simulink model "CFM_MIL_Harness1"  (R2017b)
settings: Solver=FixedStepDiscrete  StartTime=0.0  StopTime=14  FixedStep=0.01  RelTol=1e-3  EnableMultiTasking=on
undefined symbols (not defined in the file): sigbuilder_block
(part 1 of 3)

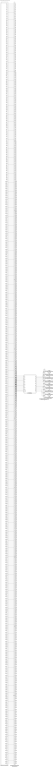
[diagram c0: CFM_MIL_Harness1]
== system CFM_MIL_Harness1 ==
  CFM_MIL : ModelReference  ModelNameDialog=CFM_MIL  SimulationMode=Normal  ModelReferenceVersion='M103C102'
  Harness Inputs : Subsystem  Tag=STV Subsys  LoadFcn=sigbuilder_block('load');  StartFcn=sigbuilder_block('start');  StopFcn=sigbuilder_block('stop');  ClipboardFcn=sigbuilder_block('clipboard');  mask(Sigbuilder block){tuvar=[0:10]}
      mask init:
      | if ~strcmp(get_param(bdroot(gcb),'SimulationStatus'),'stopped'),tuvar = sigbuilder_block('maskInit'); end
  Input Conversion Subsystem : Subsystem  Tag=__SLT_ICS__  Description=Signal spec. and routing
  Output Conversion Subsystem : Subsystem  Tag=__SLT_OCS__  Description=Signal spec. and routing
  GaCFM_AFEComLost_flg : Outport  OutDataTypeStr=boolean  PortDimensions=[8]
  GaCFM_AFECellVoltUpdErr_flg : Outport  Port=2  OutDataTypeStr=boolean  PortDimensions=[8]
  GaCFM_AFECellTempUpdErr_flg : Outport  Port=3  OutDataTypeStr=boolean  PortDimensions=[8]
  GaCFM_AFECellVoltLineOpen_flg : Outport  Port=4  OutDataTypeStr=boolean  PortDimensions=[8]
  GaCFM_AFEGpioLineOpen_flg : Outport  Port=5  OutDataTypeStr=boolean  PortDimensions=[8]
  GaCFM_AFEAdcRelatedErr_flg : Outport  Port=6  OutDataTypeStr=boolean  PortDimensions=[8]
  GaCFM_AFEDiagModeExitErr_flg : Outport  Port=7  OutDataTypeStr=boolean  PortDimensions=[8]
  GaCFM_AFEOtherErr_flg : Outport  Port=8  OutDataTypeStr=boolean  PortDimensions=[8]
  GaCFM_AFESampleErr_flg : Outport  Port=9  OutDataTypeStr=boolean  PortDimensions=[8]
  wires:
  Harness Inputs/1(GaISP_AFEComLost_numb(1)) -> Input Conversion Subsystem/1(Inport_1)
  Harness Inputs/2(GaISP_AFEComLost_numb(2)) -> Input Conversion Subsystem/2(Inport_2)
  Harness Inputs/3(GaISP_AFEComLost_numb(3)) -> Input Conversion Subsystem/3(Inport_3)
  Harness Inputs/4(GaISP_AFEComLost_numb(4)) -> Input Conversion Subsystem/4(Inport_4)
  Harness Inputs/5(GaISP_AFEComLost_numb(5)) -> Input Conversion Subsystem/5(Inport_5)
  Harness Inputs/6(GaISP_AFEComLost_numb(6)) -> Input Conversion Subsystem/6(Inport_6)
  Harness Inputs/7(GaISP_AFEComLost_numb(7)) -> Input Conversion Subsystem/7(Inport_7)
  Harness Inputs/8(GaISP_AFEComLost_numb(8)) -> Input Conversion Subsystem/8(Inport_8)
  Harness Inputs/9(GaISP_AFECellVoltUpdErr_numb(1)) -> Input Conversion Subsystem/9(Inport_9)
  Harness Inputs/10(GaISP_AFECellVoltUpdErr_numb(2)) -> Input Conversion Subsystem/10(Inport_10)
  Harness Inputs/11(GaISP_AFECellVoltUpdErr_numb(3)) -> Input Conversion Subsystem/11(Inport_11)
  Harness Inputs/12(GaISP_AFECellVoltUpdErr_numb(4)) -> Input Conversion Subsystem/12(Inport_12)
  Harness Inputs/13(GaISP_AFECellVoltUpdErr_numb(5)) -> Input Conversion Subsystem/13(Inport_13)
  Harness Inputs/14(GaISP_AFECellVoltUpdErr_numb(6)) -> Input Conversion Subsystem/14(Inport_14)
  Harness Inputs/15(GaISP_AFECellVoltUpdErr_numb(7)) -> Input Conversion Subsystem/15(Inport_15)
  Harness Inputs/16(GaISP_AFECellVoltUpdErr_numb(8)) -> Input Conversion Subsystem/16(Inport_16)
  Harness Inputs/17(GaISP_AFECellVoltUpdErr_numb(9)) -> Input Conversion Subsystem/17(Inport_17)
  Harness Inputs/18(GaISP_AFECellVoltUpdErr_numb(10)) -> Input Conversion Subsystem/18(Inport_18)
  Harness Inputs/19(GaISP_AFECellVoltUpdErr_numb(11)) -> Input Conversion Subsystem/19(Inport_19)
  Harness Inputs/20(GaISP_AFECellVoltUpdErr_numb(12)) -> Input Conversion Subsystem/20(Inport_20)
  Harness Inputs/21(GaISP_AFECellVoltUpdErr_numb(13)) -> Input Conversion Subsystem/21(Inport_21)
  Harness Inputs/22(GaISP_AFECellVoltUpdErr_numb(14)) -> Input Conversion Subsystem/22(Inport_22)
  Harness Inputs/23(GaISP_AFECellVoltUpdErr_numb(15)) -> Input Conversion Subsystem/23(Inport_23)
  Harness Inputs/24(GaISP_AFECellVoltUpdErr_numb(16)) -> Input Conversion Subsystem/24(Inport_24)
  Harness Inputs/25(GaISP_AFECellVoltUpdErr_numb(17)) -> Input Conversion Subsystem/25(Inport_25)
  Harness Inputs/26(GaISP_AFECellVoltUpdErr_numb(18)) -> Input Conversion Subsystem/26(Inport_26)
  Harness Inputs/27(GaISP_AFECellVoltUpdErr_numb(19)) -> Input Conversion Subsystem/27(Inport_27)
  Harness Inputs/28(GaISP_AFECellVoltUpdErr_numb(20)) -> Input Conversion Subsystem/28(Inport_28)
  Harness Inputs/29(GaISP_AFECellVoltUpdErr_numb(21)) -> Input Conversion Subsystem/29(Inport_29)
  Harness Inputs/30(GaISP_AFECellVoltUpdErr_numb(22)) -> Input Conversion Subsystem/30(Inport_30)
  Harness Inputs/31(GaISP_AFECellVoltUpdErr_numb(23)) -> Input Conversion Subsystem/31(Inport_31)
  Harness Inputs/32(GaISP_AFECellVoltUpdErr_numb(24)) -> Input Conversion Subsystem/32(Inport_32)
  Harness Inputs/33(GaISP_AFECellVoltUpdErr_numb(25)) -> Input Conversion Subsystem/33(Inport_33)
  Harness Inputs/34(GaISP_AFECellVoltUpdErr_numb(26)) -> Input Conversion Subsystem/34(Inport_34)
  Harness Inputs/35(GaISP_AFECellVoltUpdErr_numb(27)) -> Input Conversion Subsystem/35(Inport_35)
  Harness Inputs/36(GaISP_AFECellVoltUpdErr_numb(28)) -> Input Conversion Subsystem/36(Inport_36)
  Harness Inputs/37(GaISP_AFECellVoltUpdErr_numb(29)) -> Input Conversion Subsystem/37(Inport_37)
  Harness Inputs/38(GaISP_AFECellVoltUpdErr_numb(30)) -> Input Conversion Subsystem/38(Inport_38)
  Harness Inputs/39(GaISP_AFECellVoltUpdErr_numb(31)) -> Input Conversion Subsystem/39(Inport_39)
  Harness Inputs/40(GaISP_AFECellVoltUpdErr_numb(32)) -> Input Conversion Subsystem/40(Inport_40)
  Harness Inputs/41(GaISP_AFECellVoltUpdErr_numb(33)) -> Input Conversion Subsystem/41(Inport_41)
  Harness Inputs/42(GaISP_AFECellVoltUpdErr_numb(34)) -> Input Conversion Subsystem/42(Inport_42)
  Harness Inputs/43(GaISP_AFECellVoltUpdErr_numb(35)) -> Input Conversion Subsystem/43(Inport_43)
  Harness Inputs/44(GaISP_AFECellVoltUpdErr_numb(36)) -> Input Conversion Subsystem/44(Inport_44)
  Harness Inputs/45(GaISP_AFECellVoltUpdErr_numb(37)) -> Input Conversion Subsystem/45(Inport_45)
  Harness Inputs/46(GaISP_AFECellVoltUpdErr_numb(38)) -> Input Conversion Subsystem/46(Inport_46)
  Harness Inputs/47(GaISP_AFECellVoltUpdErr_numb(39)) -> Input Conversion Subsystem/47(Inport_47)
  Harness Inputs/48(GaISP_AFECellVoltUpdErr_numb(40)) -> Input Conversion Subsystem/48(Inport_48)
  Harness Inputs/49(GaISP_AFECellVoltUpdErr_numb(41)) -> Input Conversion Subsystem/49(Inport_49)
  Harness Inputs/50(GaISP_AFECellVoltUpdErr_numb(42)) -> Input Conversion Subsystem/50(Inport_50)
  Harness Inputs/51(GaISP_AFECellVoltUpdErr_numb(43)) -> Input Conversion Subsystem/51(Inport_51)
  Harness Inputs/52(GaISP_AFECellVoltUpdErr_numb(44)) -> Input Conversion Subsystem/52(Inport_52)
  Harness Inputs/53(GaISP_AFECellVoltUpdErr_numb(45)) -> Input Conversion Subsystem/53(Inport_53)
  Harness Inputs/54(GaISP_AFECellVoltUpdErr_numb(46)) -> Input Conversion Subsystem/54(Inport_54)
  Harness Inputs/55(GaISP_AFECellVoltUpdErr_numb(47)) -> Input Conversion Subsystem/55(Inport_55)
  Harness Inputs/56(GaISP_AFECellVoltUpdErr_numb(48)) -> Input Conversion Subsystem/56(Inport_56)
  Harness Inputs/57(GaISP_AFECellVoltUpdErr_numb(49)) -> Input Conversion Subsystem/57(Inport_57)
  Harness Inputs/58(GaISP_AFECellVoltUpdErr_numb(50)) -> Input Conversion Subsystem/58(Inport_58)
  Harness Inputs/59(GaISP_AFECellVoltUpdErr_numb(51)) -> Input Conversion Subsystem/59(Inport_59)
  Harness Inputs/60(GaISP_AFECellVoltUpdErr_numb(52)) -> Input Conversion Subsystem/60(Inport_60)
  Harness Inputs/61(GaISP_AFECellVoltUpdErr_numb(53)) -> Input Conversion Subsystem/61(Inport_61)
  Harness Inputs/62(GaISP_AFECellVoltUpdErr_numb(54)) -> Input Conversion Subsystem/62(Inport_62)
  Harness Inputs/63(GaISP_AFECellVoltUpdErr_numb(55)) -> Input Conversion Subsystem/63(Inport_63)
  Harness Inputs/64(GaISP_AFECellVoltUpdErr_numb(56)) -> Input Conversion Subsystem/64(Inport_64)
  Harness Inputs/65(GaISP_AFECellVoltUpdErr_numb(57)) -> Input Conversion Subsystem/65(Inport_65)
  Harness Inputs/66(GaISP_AFECellVoltUpdErr_numb(58)) -> Input Conversion Subsystem/66(Inport_66)
  Harness Inputs/67(GaISP_AFECellVoltUpdErr_numb(59)) -> Input Conversion Subsystem/67(Inport_67)
  Harness Inputs/68(GaISP_AFECellVoltUpdErr_numb(60)) -> Input Conversion Subsystem/68(Inport_68)
  Harness Inputs/69(GaISP_AFECellVoltUpdErr_numb(61)) -> Input Conversion Subsystem/69(Inport_69)
  Harness Inputs/70(GaISP_AFECellVoltUpdErr_numb(62)) -> Input Conversion Subsystem/70(Inport_70)
  Harness Inputs/71(GaISP_AFECellVoltUpdErr_numb(63)) -> Input Conversion Subsystem/71(Inport_71)
  Harness Inputs/72(GaISP_AFECellVoltUpdErr_numb(64)) -> Input Conversion Subsystem/72(Inport_72)
  Harness Inputs/73(GaISP_AFECellVoltUpdErr_numb(65)) -> Input Conversion Subsystem/73(Inport_73)
  Harness Inputs/74(GaISP_AFECellVoltUpdErr_numb(66)) -> Input Conversion Subsystem/74(Inport_74)
  Harness Inputs/75(GaISP_AFECellVoltUpdErr_numb(67)) -> Input Conversion Subsystem/75(Inport_75)
  Harness Inputs/76(GaISP_AFECellVoltUpdErr_numb(68)) -> Input Conversion Subsystem/76(Inport_76)
  Harness Inputs/77(GaISP_AFECellVoltUpdErr_numb(69)) -> Input Conversion Subsystem/77(Inport_77)
  Harness Inputs/78(GaISP_AFECellVoltUpdErr_numb(70)) -> Input Conversion Subsystem/78(Inport_78)
  Harness Inputs/79(GaISP_AFECellVoltUpdErr_numb(71)) -> Input Conversion Subsystem/79(Inport_79)
  Harness Inputs/80(GaISP_AFECellVoltUpdErr_numb(72)) -> Input Conversion Subsystem/80(Inport_80)
  Harness Inputs/81(GaISP_AFECellVoltUpdErr_numb(73)) -> Input Conversion Subsystem/81(Inport_81)
  Harness Inputs/82(GaISP_AFECellVoltUpdErr_numb(74)) -> Input Conversion Subsystem/82(Inport_82)
  Harness Inputs/83(GaISP_AFECellVoltUpdErr_numb(75)) -> Input Conversion Subsystem/83(Inport_83)
  Harness Inputs/84(GaISP_AFECellVoltUpdErr_numb(76)) -> Input Conversion Subsystem/84(Inport_84)
  Harness Inputs/85(GaISP_AFECellVoltUpdErr_numb(77)) -> Input Conversion Subsystem/85(Inport_85)
  Harness Inputs/86(GaISP_AFECellVoltUpdErr_numb(78)) -> Input Conversion Subsystem/86(Inport_86)
  Harness Inputs/87(GaISP_AFECellVoltUpdErr_numb(79)) -> Input Conversion Subsystem/87(Inport_87)
  Harness Inputs/88(GaISP_AFECellVoltUpdErr_numb(80)) -> Input Conversion Subsystem/88(Inport_88)
  Harness Inputs/89(GaISP_AFECellVoltUpdErr_numb(81)) -> Input Conversion Subsystem/89(Inport_89)
  Harness Inputs/90(GaISP_AFECellVoltUpdErr_numb(82)) -> Input Conversion Subsystem/90(Inport_90)
  Harness Inputs/91(GaISP_AFECellVoltUpdErr_numb(83)) -> Input Conversion Subsystem/91(Inport_91)
  Harness Inputs/92(GaISP_AFECellVoltUpdErr_numb(84)) -> Input Conversion Subsystem/92(Inport_92)
  Harness Inputs/93(GaISP_AFECellVoltUpdErr_numb(85)) -> Input Conversion Subsystem/93(Inport_93)
  Harness Inputs/94(GaISP_AFECellVoltUpdErr_numb(86)) -> Input Conversion Subsystem/94(Inport_94)
  Harness Inputs/95(GaISP_AFECellVoltUpdErr_numb(87)) -> Input Conversion Subsystem/95(Inport_95)
  Harness Inputs/96(GaISP_AFECellVoltUpdErr_numb(88)) -> Input Conversion Subsystem/96(Inport_96)
  Harness Inputs/97(GaISP_AFECellVoltUpdErr_numb(89)) -> Input Conversion Subsystem/97(Inport_97)
  Harness Inputs/98(GaISP_AFECellVoltUpdErr_numb(90)) -> Input Conversion Subsystem/98(Inport_98)
  Harness Inputs/99(GaISP_AFECellVoltUpdErr_numb(91)) -> Input Conversion Subsystem/99(Inport_99)
  Harness Inputs/100(GaISP_AFECellVoltUpdErr_numb(92)) -> Input Conversion Subsystem/100(Inport_100)
  Harness Inputs/101(GaISP_AFECellVoltUpdErr_numb(93)) -> Input Conversion Subsystem/101(Inport_101)
  Harness Inputs/102(GaISP_AFECellVoltUpdErr_numb(94)) -> Input Conversion Subsystem/102(Inport_102)
  Harness Inputs/103(GaISP_AFECellVoltUpdErr_numb(95)) -> Input Conversion Subsystem/103(Inport_103)
  Harness Inputs/104(GaISP_AFECellVoltUpdErr_numb(96)) -> Input Conversion Subsystem/104(Inport_104)
  Harness Inputs/105(GaISP_AFECellVoltUpdErr_numb(97)) -> Input Conversion Subsystem/105(Inport_105)
  Harness Inputs/106(GaISP_AFECellVoltUpdErr_numb(98)) -> Input Conversion Subsystem/106(Inport_106)
  Harness Inputs/107(GaISP_AFECellVoltUpdErr_numb(99)) -> Input Conversion Subsystem/107(Inport_107)
  Harness Inputs/108(GaISP_AFECellVoltUpdErr_numb(100)) -> Input Conversion Subsystem/108(Inport_108)
  Harness Inputs/109(GaISP_AFECellVoltUpdErr_numb(101)) -> Input Conversion Subsystem/109(Inport_109)
  Harness Inputs/110(GaISP_AFECellVoltUpdErr_numb(102)) -> Input Conversion Subsystem/110(Inport_110)
  Harness Inputs/111(GaISP_AFECellVoltUpdErr_numb(103)) -> Input Conversion Subsystem/111(Inport_111)
  Harness Inputs/112(GaISP_AFECellVoltUpdErr_numb(104)) -> Input Conversion Subsystem/112(Inport_112)
  Harness Inputs/113(GaISP_AFECellVoltUpdErr_numb(105)) -> Input Conversion Subsystem/113(Inport_113)
  Harness Inputs/114(GaISP_AFECellVoltUpdErr_numb(106)) -> Input Conversion Subsystem/114(Inport_114)
  Harness Inputs/115(GaISP_AFECellVoltUpdErr_numb(107)) -> Input Conversion Subsystem/115(Inport_115)
  Harness Inputs/116(GaISP_AFECellVoltUpdErr_numb(108)) -> Input Conversion Subsystem/116(Inport_116)
  Harness Inputs/117(GaISP_AFECellVoltUpdErr_numb(109)) -> Input Conversion Subsystem/117(Inport_117)
  Harness Inputs/118(GaISP_AFECellVoltUpdErr_numb(110)) -> Input Conversion Subsystem/118(Inport_118)
  Harness Inputs/119(GaISP_AFECellVoltUpdErr_numb(111)) -> Input Conversion Subsystem/119(Inport_119)
  Harness Inputs/120(GaISP_AFECellVoltUpdErr_numb(112)) -> Input Conversion Subsystem/120(Inport_120)
  Harness Inputs/121(GaISP_AFECellTempUpdErr_numb(1)) -> Input Conversion Subsystem/121(Inport_121)
  Harness Inputs/122(GaISP_AFECellTempUpdErr_numb(2)) -> Input Conversion Subsystem/122(Inport_122)
  Harness Inputs/123(GaISP_AFECellTempUpdErr_numb(3)) -> Input Conversion Subsystem/123(Inport_123)
  Harness Inputs/124(GaISP_AFECellTempUpdErr_numb(4)) -> Input Conversion Subsystem/124(Inport_124)
  Harness Inputs/125(GaISP_AFECellTempUpdErr_numb(5)) -> Input Conversion Subsystem/125(Inport_125)
  Harness Inputs/126(GaISP_AFECellTempUpdErr_numb(6)) -> Input Conversion Subsystem/126(Inport_126)
  Harness Inputs/127(GaISP_AFECellTempUpdErr_numb(7)) -> Input Conversion Subsystem/127(Inport_127)
  Harness Inputs/128(GaISP_AFECellTempUpdErr_numb(8)) -> Input Conversion Subsystem/128(Inport_128)
  Harness Inputs/129(GaISP_AFECellTempUpdErr_numb(9)) -> Input Conversion Subsystem/129(Inport_129)
  Harness Inputs/130(GaISP_AFECellTempUpdErr_numb(10)) -> Input Conversion Subsystem/130(Inport_130)
  Harness Inputs/131(GaISP_AFECellTempUpdErr_numb(11)) -> Input Conversion Subsystem/131(Inport_131)
  Harness Inputs/132(GaISP_AFECellTempUpdErr_numb(12)) -> Input Conversion Subsystem/132(Inport_132)
  Harness Inputs/133(GaISP_AFECellTempUpdErr_numb(13)) -> Input Conversion Subsystem/133(Inport_133)
  Harness Inputs/134(GaISP_AFECellTempUpdErr_numb(14)) -> Input Conversion Subsystem/134(Inport_134)
  Harness Inputs/135(GaISP_AFECellTempUpdErr_numb(15)) -> Input Conversion Subsystem/135(Inport_135)
  Harness Inputs/136(GaISP_AFECellTempUpdErr_numb(16)) -> Input Conversion Subsystem/136(Inport_136)
  Harness Inputs/137(GaISP_AFECellTempUpdErr_numb(17)) -> Input Conversion Subsystem/137(Inport_137)
  Harness Inputs/138(GaISP_AFECellTempUpdErr_numb(18)) -> Input Conversion Subsystem/138(Inport_138)
  Harness Inputs/139(GaISP_AFECellTempUpdErr_numb(19)) -> Input Conversion Subsystem/139(Inport_139)
  Harness Inputs/140(GaISP_AFECellTempUpdErr_numb(20)) -> Input Conversion Subsystem/140(Inport_140)
  Harness Inputs/141(GaISP_AFECellTempUpdErr_numb(21)) -> Input Conversion Subsystem/141(Inport_141)
  Harness Inputs/142(GaISP_AFECellTempUpdErr_numb(22)) -> Input Conversion Subsystem/142(Inport_142)
  Harness Inputs/143(GaISP_AFECellTempUpdErr_numb(23)) -> Input Conversion Subsystem/143(Inport_143)
  Harness Inputs/144(GaISP_AFECellTempUpdErr_numb(24)) -> Input Conversion Subsystem/144(Inport_144)
  Harness Inputs/145(GaISP_AFECellTempUpdErr_numb(25)) -> Input Conversion Subsystem/145(Inport_145)
  Harness Inputs/146(GaISP_AFECellTempUpdErr_numb(26)) -> Input Conversion Subsystem/146(Inport_146)
  Harness Inputs/147(GaISP_AFECellTempUpdErr_numb(27)) -> Input Conversion Subsystem/147(Inport_147)
  Harness Inputs/148(GaISP_AFECellTempUpdErr_numb(28)) -> Input Conversion Subsystem/148(Inport_148)
  Harness Inputs/149(GaISP_AFECellTempUpdErr_numb(29)) -> Input Conversion Subsystem/149(Inport_149)
  Harness Inputs/150(GaISP_AFECellTempUpdErr_numb(30)) -> Input Conversion Subsystem/150(Inport_150)
  Harness Inputs/151(GaISP_AFECellTempUpdErr_numb(31)) -> Input Conversion Subsystem/151(Inport_151)
  Harness Inputs/152(GaISP_AFECellTempUpdErr_numb(32)) -> Input Conversion Subsystem/152(Inport_152)
  Harness Inputs/153(GaISP_AFECellTempUpdErr_numb(33)) -> Input Conversion Subsystem/153(Inport_153)
  Harness Inputs/154(GaISP_AFECellTempUpdErr_numb(34)) -> Input Conversion Subsystem/154(Inport_154)
  Harness Inputs/155(GaISP_AFECellTempUpdErr_numb(35)) -> Input Conversion Subsystem/155(Inport_155)
  Harness Inputs/156(GaISP_AFECellTempUpdErr_numb(36)) -> Input Conversion Subsystem/156(Inport_156)
  Harness Inputs/157(GaISP_AFECellTempUpdErr_numb(37)) -> Input Conversion Subsystem/157(Inport_157)
  Harness Inputs/158(GaISP_AFECellTempUpdErr_numb(38)) -> Input Conversion Subsystem/158(Inport_158)
  Harness Inputs/159(GaISP_AFECellTempUpdErr_numb(39)) -> Input Conversion Subsystem/159(Inport_159)
  Harness Inputs/160(GaISP_AFECellTempUpdErr_numb(40)) -> Input Conversion Subsystem/160(Inport_160)
  Harness Inputs/161(GaISP_AFECellTempUpdErr_numb(41)) -> Input Conversion Subsystem/161(Inport_161)
  Harness Inputs/162(GaISP_AFECellTempUpdErr_numb(42)) -> Input Conversion Subsystem/162(Inport_162)
  Harness Inputs/163(GaISP_AFECellTempUpdErr_numb(43)) -> Input Conversion Subsystem/163(Inport_163)
  Harness Inputs/164(GaISP_AFECellTempUpdErr_numb(44)) -> Input Conversion Subsystem/164(Inport_164)
  Harness Inputs/165(GaISP_AFECellTempUpdErr_numb(45)) -> Input Conversion Subsystem/165(Inport_165)
  Harness Inputs/166(GaISP_AFECellTempUpdErr_numb(46)) -> Input Conversion Subsystem/166(Inport_166)
  Harness Inputs/167(GaISP_AFECellTempUpdErr_numb(47)) -> Input Conversion Subsystem/167(Inport_167)
  Harness Inputs/168(GaISP_AFECellTempUpdErr_numb(48)) -> Input Conversion Subsystem/168(Inport_168)
  Harness Inputs/169(GaISP_AFECellVoltLineOpen_numb(1)) -> Input Conversion Subsystem/169(Inport_169)
  Harness Inputs/170(GaISP_AFECellVoltLineOpen_numb(2)) -> Input Conversion Subsystem/170(Inport_170)
  Harness Inputs/171(GaISP_AFECellVoltLineOpen_numb(3)) -> Input Conversion Subsystem/171(Inport_171)
  Harness Inputs/172(GaISP_AFECellVoltLineOpen_numb(4)) -> Input Conversion Subsystem/172(Inport_172)
  Harness Inputs/173(GaISP_AFECellVoltLineOpen_numb(5)) -> Input Conversion Subsystem/173(Inport_173)
  Harness Inputs/174(GaISP_AFECellVoltLineOpen_numb(6)) -> Input Conversion Subsystem/174(Inport_174)
  Harness Inputs/175(GaISP_AFECellVoltLineOpen_numb(7)) -> Input Conversion Subsystem/175(Inport_175)
  Harness Inputs/176(GaISP_AFECellVoltLineOpen_numb(8)) -> Input Conversion Subsystem/176(Inport_176)
  Harness Inputs/177(GaISP_AFECellVoltLineOpen_numb(9)) -> Input Conversion Subsystem/177(Inport_177)
  Harness Inputs/178(GaISP_AFECellVoltLineOpen_numb(10)) -> Input Conversion Subsystem/178(Inport_178)
  Harness Inputs/179(GaISP_AFECellVoltLineOpen_numb(11)) -> Input Conversion Subsystem/179(Inport_179)
  Harness Inputs/180(GaISP_AFECellVoltLineOpen_numb(12)) -> Input Conversion Subsystem/180(Inport_180)
  Harness Inputs/181(GaISP_AFECellVoltLineOpen_numb(13)) -> Input Conversion Subsystem/181(Inport_181)
  Harness Inputs/182(GaISP_AFECellVoltLineOpen_numb(14)) -> Input Conversion Subsystem/182(Inport_182)
  Harness Inputs/183(GaISP_AFECellVoltLineOpen_numb(15)) -> Input Conversion Subsystem/183(Inport_183)
  Harness Inputs/184(GaISP_AFECellVoltLineOpen_numb(16)) -> Input Conversion Subsystem/184(Inport_184)
  Harness Inputs/185(GaISP_AFECellVoltLineOpen_numb(17)) -> Input Conversion Subsystem/185(Inport_185)
  Harness Inputs/186(GaISP_AFECellVoltLineOpen_numb(18)) -> Input Conversion Subsystem/186(Inport_186)
  Harness Inputs/187(GaISP_AFECellVoltLineOpen_numb(19)) -> Input Conversion Subsystem/187(Inport_187)
  Harness Inputs/188(GaISP_AFECellVoltLineOpen_numb(20)) -> Input Conversion Subsystem/188(Inport_188)
  Harness Inputs/189(GaISP_AFECellVoltLineOpen_numb(21)) -> Input Conversion Subsystem/189(Inport_189)
  Harness Inputs/190(GaISP_AFECellVoltLineOpen_numb(22)) -> Input Conversion Subsystem/190(Inport_190)
  Harness Inputs/191(GaISP_AFECellVoltLineOpen_numb(23)) -> Input Conversion Subsystem/191(Inport_191)
  Harness Inputs/192(GaISP_AFECellVoltLineOpen_numb(24)) -> Input Conversion Subsystem/192(Inport_192)
  Harness Inputs/193(GaISP_AFECellVoltLineOpen_numb(25)) -> Input Conversion Subsystem/193(Inport_193)
  Harness Inputs/194(GaISP_AFECellVoltLineOpen_numb(26)) -> Input Conversion Subsystem/194(Inport_194)
  Harness Inputs/195(GaISP_AFECellVoltLineOpen_numb(27)) -> Input Conversion Subsystem/195(Inport_195)
  Harness Inputs/196(GaISP_AFECellVoltLineOpen_numb(28)) -> Input Conversion Subsystem/196(Inport_196)
  Harness Inputs/197(GaISP_AFECellVoltLineOpen_numb(29)) -> Input Conversion Subsystem/197(Inport_197)
  Harness Inputs/198(GaISP_AFECellVoltLineOpen_numb(30)) -> Input Conversion Subsystem/198(Inport_198)
  Harness Inputs/199(GaISP_AFECellVoltLineOpen_numb(31)) -> Input Conversion Subsystem/199(Inport_199)
  Harness Inputs/200(GaISP_AFECellVoltLineOpen_numb(32)) -> Input Conversion Subsystem/200(Inport_200)
  Harness Inputs/201(GaISP_AFECellVoltLineOpen_numb(33)) -> Input Conversion Subsystem/201(Inport_201)
  Harness Inputs/202(GaISP_AFECellVoltLineOpen_numb(34)) -> Input Conversion Subsystem/202(Inport_202)
  Harness Inputs/203(GaISP_AFECellVoltLineOpen_numb(35)) -> Input Conversion Subsystem/203(Inport_203)
  Harness Inputs/204(GaISP_AFECellVoltLineOpen_numb(36)) -> Input Conversion Subsystem/204(Inport_204)
  Harness Inputs/205(GaISP_AFECellVoltLineOpen_numb(37)) -> Input Conversion Subsystem/205(Inport_205)
  Harness Inputs/206(GaISP_AFECellVoltLineOpen_numb(38)) -> Input Conversion Subsystem/206(Inport_206)
  Harness Inputs/207(GaISP_AFECellVoltLineOpen_numb(39)) -> Input Conversion Subsystem/207(Inport_207)
  Harness Inputs/208(GaISP_AFECellVoltLineOpen_numb(40)) -> Input Conversion Subsystem/208(Inport_208)
  Harness Inputs/209(GaISP_AFECellVoltLineOpen_numb(41)) -> Input Conversion Subsystem/209(Inport_209)
  Harness Inputs/210(GaISP_AFECellVoltLineOpen_numb(42)) -> Input Conversion Subsystem/210(Inport_210)
  Harness Inputs/211(GaISP_AFECellVoltLineOpen_numb(43)) -> Input Conversion Subsystem/211(Inport_211)
  Harness Inputs/212(GaISP_AFECellVoltLineOpen_numb(44)) -> Input Conversion Subsystem/212(Inport_212)
  Harness Inputs/213(GaISP_AFECellVoltLineOpen_numb(45)) -> Input Conversion Subsystem/213(Inport_213)
  Harness Inputs/214(GaISP_AFECellVoltLineOpen_numb(46)) -> Input Conversion Subsystem/214(Inport_214)
  Harness Inputs/215(GaISP_AFECellVoltLineOpen_numb(47)) -> Input Conversion Subsystem/215(Inport_215)
  Harness Inputs/216(GaISP_AFECellVoltLineOpen_numb(48)) -> Input Conversion Subsystem/216(Inport_216)
  Harness Inputs/217(GaISP_AFECellVoltLineOpen_numb(49)) -> Input Conversion Subsystem/217(Inport_217)
  Harness Inputs/218(GaISP_AFECellVoltLineOpen_numb(50)) -> Input Conversion Subsystem/218(Inport_218)
  Harness Inputs/219(GaISP_AFECellVoltLineOpen_numb(51)) -> Input Conversion Subsystem/219(Inport_219)
  Harness Inputs/220(GaISP_AFECellVoltLineOpen_numb(52)) -> Input Conversion Subsystem/220(Inport_220)
  Harness Inputs/221(GaISP_AFECellVoltLineOpen_numb(53)) -> Input Conversion Subsystem/221(Inport_221)
  Harness Inputs/222(GaISP_AFECellVoltLineOpen_numb(54)) -> Input Conversion Subsystem/222(Inport_222)
  Harness Inputs/223(GaISP_AFECellVoltLineOpen_numb(55)) -> Input Conversion Subsystem/223(Inport_223)
  Harness Inputs/224(GaISP_AFECellVoltLineOpen_numb(56)) -> Input Conversion Subsystem/224(Inport_224)
  Harness Inputs/225(GaISP_AFECellVoltLineOpen_numb(57)) -> Input Conversion Subsystem/225(Inport_225)
  Harness Inputs/226(GaISP_AFECellVoltLineOpen_numb(58)) -> Input Conversion Subsystem/226(Inport_226)
  Harness Inputs/227(GaISP_AFECellVoltLineOpen_numb(59)) -> Input Conversion Subsystem/227(Inport_227)
  Harness Inputs/228(GaISP_AFECellVoltLineOpen_numb(60)) -> Input Conversion Subsystem/228(Inport_228)
  Harness Inputs/229(GaISP_AFECellVoltLineOpen_numb(61)) -> Input Conversion Subsystem/229(Inport_229)
  Harness Inputs/230(GaISP_AFECellVoltLineOpen_numb(62)) -> Input Conversion Subsystem/230(Inport_230)
  Harness Inputs/231(GaISP_AFECellVoltLineOpen_numb(63)) -> Input Conversion Subsystem/231(Inport_231)
  Harness Inputs/232(GaISP_AFECellVoltLineOpen_numb(64)) -> Input Conversion Subsystem/232(Inport_232)
  Harness Inputs/233(GaISP_AFECellVoltLineOpen_numb(65)) -> Input Conversion Subsystem/233(Inport_233)
  Harness Inputs/234(GaISP_AFECellVoltLineOpen_numb(66)) -> Input Conversion Subsystem/234(Inport_234)
  Harness Inputs/235(GaISP_AFECellVoltLineOpen_numb(67)) -> Input Conversion Subsystem/235(Inport_235)
  Harness Inputs/236(GaISP_AFECellVoltLineOpen_numb(68)) -> Input Conversion Subsystem/236(Inport_236)
  Harness Inputs/237(GaISP_AFECellVoltLineOpen_numb(69)) -> Input Conversion Subsystem/237(Inport_237)
  Harness Inputs/238(GaISP_AFECellVoltLineOpen_numb(70)) -> Input Conversion Subsystem/238(Inport_238)
  Harness Inputs/239(GaISP_AFECellVoltLineOpen_numb(71)) -> Input Conversion Subsystem/239(Inport_239)
  Harness Inputs/240(GaISP_AFECellVoltLineOpen_numb(72)) -> Input Conversion Subsystem/240(Inport_240)
  Harness Inputs/241(GaISP_AFECellVoltLineOpen_numb(73)) -> Input Conversion Subsystem/241(Inport_241)
  Harness Inputs/242(GaISP_AFECellVoltLineOpen_numb(74)) -> Input Conversion Subsystem/242(Inport_242)
  Harness Inputs/243(GaISP_AFECellVoltLineOpen_numb(75)) -> Input Conversion Subsystem/243(Inport_243)
  Harness Inputs/244(GaISP_AFECellVoltLineOpen_numb(76)) -> Input Conversion Subsystem/244(Inport_244)
  Harness Inputs/245(GaISP_AFECellVoltLineOpen_numb(77)) -> Input Conversion Subsystem/245(Inport_245)
  Harness Inputs/246(GaISP_AFECellVoltLineOpen_numb(78)) -> Input Conversion Subsystem/246(Inport_246)
  Harness Inputs/247(GaISP_AFECellVoltLineOpen_numb(79)) -> Input Conversion Subsystem/247(Inport_247)
  Harness Inputs/248(GaISP_AFECellVoltLineOpen_numb(80)) -> Input Conversion Subsystem/248(Inport_248)
  Harness Inputs/249(GaISP_AFECellVoltLineOpen_numb(81)) -> Input Conversion Subsystem/249(Inport_249)
  Harness Inputs/250(GaISP_AFECellVoltLineOpen_numb(82)) -> Input Conversion Subsystem/250(Inport_250)
  Harness Inputs/251(GaISP_AFECellVoltLineOpen_numb(83)) -> Input Conversion Subsystem/251(Inport_251)
  Harness Inputs/252(GaISP_AFECellVoltLineOpen_numb(84)) -> Input Conversion Subsystem/252(Inport_252)
  Harness Inputs/253(GaISP_AFECellVoltLineOpen_numb(85)) -> Input Conversion Subsystem/253(Inport_253)
  Harness Inputs/254(GaISP_AFECellVoltLineOpen_numb(86)) -> Input Conversion Subsystem/254(Inport_254)
  Harness Inputs/255(GaISP_AFECellVoltLineOpen_numb(87)) -> Input Conversion Subsystem/255(Inport_255)
  Harness Inputs/256(GaISP_AFECellVoltLineOpen_numb(88)) -> Input Conversion Subsystem/256(Inport_256)
  Harness Inputs/257(GaISP_AFECellVoltLineOpen_numb(89)) -> Input Conversion Subsystem/257(Inport_257)
  Harness Inputs/258(GaISP_AFECellVoltLineOpen_numb(90)) -> Input Conversion Subsystem/258(Inport_258)
  Harness Inputs/259(GaISP_AFECellVoltLineOpen_numb(91)) -> Input Conversion Subsystem/259(Inport_259)
  Harness Inputs/260(GaISP_AFECellVoltLineOpen_numb(92)) -> Input Conversion Subsystem/260(Inport_260)
  Harness Inputs/261(GaISP_AFECellVoltLineOpen_numb(93)) -> Input Conversion Subsystem/261(Inport_261)
  Harness Inputs/262(GaISP_AFECellVoltLineOpen_numb(94)) -> Input Conversion Subsystem/262(Inport_262)
  Harness Inputs/263(GaISP_AFECellVoltLineOpen_numb(95)) -> Input Conversion Subsystem/263(Inport_263)
  Harness Inputs/264(GaISP_AFECellVoltLineOpen_numb(96)) -> Input Conversion Subsystem/264(Inport_264)
  Harness Inputs/265(GaISP_AFECellVoltLineOpen_numb(97)) -> Input Conversion Subsystem/265(Inport_265)
  Harness Inputs/266(GaISP_AFECellVoltLineOpen_numb(98)) -> Input Conversion Subsystem/266(Inport_266)
  Harness Inputs/267(GaISP_AFECellVoltLineOpen_numb(99)) -> Input Conversion Subsystem/267(Inport_267)
  Harness Inputs/268(GaISP_AFECellVoltLineOpen_numb(100)) -> Input Conversion Subsystem/268(Inport_268)
  Harness Inputs/269(GaISP_AFECellVoltLineOpen_numb(101)) -> Input Conversion Subsystem/269(Inport_269)
  Harness Inputs/270(GaISP_AFECellVoltLineOpen_numb(102)) -> Input Conversion Subsystem/270(Inport_270)
  Harness Inputs/271(GaISP_AFECellVoltLineOpen_numb(103)) -> Input Conversion Subsystem/271(Inport_271)
  Harness Inputs/272(GaISP_AFECellVoltLineOpen_numb(104)) -> Input Conversion Subsystem/272(Inport_272)
  Harness Inputs/273(GaISP_AFECellVoltLineOpen_numb(105)) -> Input Conversion Subsystem/273(Inport_273)
  Harness Inputs/274(GaISP_AFECellVoltLineOpen_numb(106)) -> Input Conversion Subsystem/274(Inport_274)
  Harness Inputs/275(GaISP_AFECellVoltLineOpen_numb(107)) -> Input Conversion Subsystem/275(Inport_275)
  Harness Inputs/276(GaISP_AFECellVoltLineOpen_numb(108)) -> Input Conversion Subsystem/276(Inport_276)
  Harness Inputs/277(GaISP_AFECellVoltLineOpen_numb(109)) -> Input Conversion Subsystem/277(Inport_277)
  Harness Inputs/278(GaISP_AFECellVoltLineOpen_numb(110)) -> Input Conversion Subsystem/278(Inport_278)
  Harness Inputs/279(GaISP_AFECellVoltLineOpen_numb(111)) -> Input Conversion Subsystem/279(Inport_279)
  Harness Inputs/280(GaISP_AFECellVoltLineOpen_numb(112)) -> Input Conversion Subsystem/280(Inport_280)
  Harness Inputs/281(GaCDP_AFETempSampAbn_flg(1)) -> Input Conversion Subsystem/281(Inport_281)
  Harness Inputs/282(GaCDP_AFETempSampAbn_flg(2)) -> Input Conversion Subsystem/282(Inport_282)
  Harness Inputs/283(GaCDP_AFETempSampAbn_flg(3)) -> Input Conversion Subsystem/283(Inport_283)
  Harness Inputs/284(GaCDP_AFETempSampAbn_flg(4)) -> Input Conversion Subsystem/284(Inport_284)
  Harness Inputs/285(GaCDP_AFETempSampAbn_flg(5)) -> Input Conversion Subsystem/285(Inport_285)
  Harness Inputs/286(GaCDP_AFETempSampAbn_flg(6)) -> Input Conversion Subsystem/286(Inport_286)
  Harness Inputs/287(GaCDP_AFETempSampAbn_flg(7)) -> Input Conversion Subsystem/287(Inport_287)
  Harness Inputs/288(GaCDP_AFETempSampAbn_flg(8)) -> Input Conversion Subsystem/288(Inport_288)
  Harness Inputs/289(GaISP_AFEAdcRelatedErr_numb(1)) -> Input Conversion Subsystem/289(Inport_289)
  Harness Inputs/290(GaISP_AFEAdcRelatedErr_numb(2)) -> Input Conversion Subsystem/290(Inport_290)
  Harness Inputs/291(GaISP_AFEAdcRelatedErr_numb(3)) -> Input Conversion Subsystem/291(Inport_291)
  Harness Inputs/292(GaISP_AFEAdcRelatedErr_numb(4)) -> Input Conversion Subsystem/292(Inport_292)
  Harness Inputs/293(GaISP_AFEAdcRelatedErr_numb(5)) -> Input Conversion Subsystem/293(Inport_293)
  Harness Inputs/294(GaISP_AFEAdcRelatedErr_numb(6)) -> Input Conversion Subsystem/294(Inport_294)
  Harness Inputs/295(GaISP_AFEAdcRelatedErr_numb(7)) -> Input Conversion Subsystem/295(Inport_295)
  Harness Inputs/296(GaISP_AFEAdcRelatedErr_numb(8)) -> Input Conversion Subsystem/296(Inport_296)
  Harness Inputs/297(GaISP_AFEAdcRelatedErr_numb(9)) -> Input Conversion Subsystem/297(Inport_297)
  Harness Inputs/298(GaISP_AFEAdcRelatedErr_numb(10)) -> Input Conversion Subsystem/298(Inport_298)
  Harness Inputs/299(GaISP_AFEAdcRelatedErr_numb(11)) -> Input Conversion Subsystem/299(Inport_299)
  Harness Inputs/300(GaISP_AFEAdcRelatedErr_numb(12)) -> Input Conversion Subsystem/300(Inport_300)
  Harness Inputs/301(GaISP_AFEAdcRelatedErr_numb(13)) -> Input Conversion Subsystem/301(Inport_301)
  Harness Inputs/302(GaISP_AFEAdcRelatedErr_numb(14)) -> Input Conversion Subsystem/302(Inport_302)
  Harness Inputs/303(GaISP_AFEAdcRelatedErr_numb(15)) -> Input Conversion Subsystem/303(Inport_303)
  Harness Inputs/304(GaISP_AFEAdcRelatedErr_numb(16)) -> Input Conversion Subsystem/304(Inport_304)
  Harness Inputs/305(GaISP_AFEAdcRelatedErr_numb(17)) -> Input Conversion Subsystem/305(Inport_305)
  Harness Inputs/306(GaISP_AFEAdcRelatedErr_numb(18)) -> Input Conversion Subsystem/306(Inport_306)
  Harness Inputs/307(GaISP_AFEAdcRelatedErr_numb(19)) -> Input Conversion Subsystem/307(Inport_307)
  Harness Inputs/308(GaISP_AFEAdcRelatedErr_numb(20)) -> Input Conversion Subsystem/308(Inport_308)
  Harness Inputs/309(GaISP_AFEAdcRelatedErr_numb(21)) -> Input Conversion Subsystem/309(Inport_309)
  Harness Inputs/310(GaISP_AFEAdcRelatedErr_numb(22)) -> Input Conversion Subsystem/310(Inport_310)
  Harness Inputs/311(GaISP_AFEAdcRelatedErr_numb(23)) -> Input Conversion Subsystem/311(Inport_311)
  Harness Inputs/312(GaISP_AFEAdcRelatedErr_numb(24)) -> Input Conversion Subsystem/312(Inport_312)
  Harness Inputs/313(GaISP_AFEAdcRelatedErr_numb(25)) -> Input Conversion Subsystem/313(Inport_313)
  Harness Inputs/314(GaISP_AFEAdcRelatedErr_numb(26)) -> Input Conversion Subsystem/314(Inport_314)
  Harness Inputs/315(GaISP_AFEAdcRelatedErr_numb(27)) -> Input Conversion Subsystem/315(Inport_315)
  Harness Inputs/316(GaISP_AFEAdcRelatedErr_numb(28)) -> Input Conversion Subsystem/316(Inport_316)
  Harness Inputs/317(GaISP_AFEAdcRelatedErr_numb(29)) -> Input Conversion Subsystem/317(Inport_317)
  Harness Inputs/318(GaISP_AFEAdcRelatedErr_numb(30)) -> Input Conversion Subsystem/318(Inport_318)
  Harness Inputs/319(GaISP_AFEAdcRelatedErr_numb(31)) -> Input Conversion Subsystem/319(Inport_319)
  Harness Inputs/320(GaISP_AFEAdcRelatedErr_numb(32)) -> Input Conversion Subsystem/320(Inport_320)
  Harness Inputs/321(GaISP_AFEAdcRelatedErr_numb(33)) -> Input Conversion Subsystem/321(Inport_321)
  Harness Inputs/322(GaISP_AFEAdcRelatedErr_numb(34)) -> Input Conversion Subsystem/322(Inport_322)
  Harness Inputs/323(GaISP_AFEAdcRelatedErr_numb(35)) -> Input Conversion Subsystem/323(Inport_323)
  Harness Inputs/324(GaISP_AFEAdcRelatedErr_numb(36)) -> Input Conversion Subsystem/324(Inport_324)
  Harness Inputs/325(GaISP_AFEAdcRelatedErr_numb(37)) -> Input Conversion Subsystem/325(Inport_325)
  Harness Inputs/326(GaISP_AFEAdcRelatedErr_numb(38)) -> Input Conversion Subsystem/326(Inport_326)
  Harness Inputs/327(GaISP_AFEAdcRelatedErr_numb(39)) -> Input Conversion Subsystem/327(Inport_327)
  Harness Inputs/328(GaISP_AFEAdcRelatedErr_numb(40)) -> Input Conversion Subsystem/328(Inport_328)
  Harness Inputs/329(GaISP_AFEAdcRelatedErr_numb(41)) -> Input Conversion Subsystem/329(Inport_329)
  Harness Inputs/330(GaISP_AFEAdcRelatedErr_numb(42)) -> Input Conversion Subsystem/330(Inport_330)
  Harness Inputs/331(GaISP_AFEAdcRelatedErr_numb(43)) -> Input Conversion Subsystem/331(Inport_331)
  Harness Inputs/332(GaISP_AFEAdcRelatedErr_numb(44)) -> Input Conversion Subsystem/332(Inport_332)
  Harness Inputs/333(GaISP_AFEAdcRelatedErr_numb(45)) -> Input Conversion Subsystem/333(Inport_333)
  Harness Inputs/334(GaISP_AFEAdcRelatedErr_numb(46)) -> Input Conversion Subsystem/334(Inport_334)
  Harness Inputs/335(GaISP_AFEAdcRelatedErr_numb(47)) -> Input Conversion Subsystem/335(Inport_335)
  Harness Inputs/336(GaISP_AFEAdcRelatedErr_numb(48)) -> Input Conversion Subsystem/336(Inport_336)
  Harness Inputs/337(GaISP_AFEAdcRelatedErr_numb(49)) -> Input Conversion Subsystem/337(Inport_337)
  Harness Inputs/338(GaISP_AFEAdcRelatedErr_numb(50)) -> Input Conversion Subsystem/338(Inport_338)
  Harness Inputs/339(GaISP_AFEAdcRelatedErr_numb(51)) -> Input Conversion Subsystem/339(Inport_339)
  Harness Inputs/340(GaISP_AFEAdcRelatedErr_numb(52)) -> Input Conversion Subsystem/340(Inport_340)
  Harness Inputs/341(GaISP_AFEAdcRelatedErr_numb(53)) -> Input Conversion Subsystem/341(Inport_341)
  Harness Inputs/342(GaISP_AFEAdcRelatedErr_numb(54)) -> Input Conversion Subsystem/342(Inport_342)
  Harness Inputs/343(GaISP_AFEAdcRelatedErr_numb(55)) -> Input Conversion Subsystem/343(Inport_343)
  Harness Inputs/344(GaISP_AFEAdcRelatedErr_numb(56)) -> Input Conversion Subsystem/344(Inport_344)
  Harness Inputs/345(GaISP_AFEAdcRelatedErr_numb(57)) -> Input Conversion Subsystem/345(Inport_345)
  Harness Inputs/346(GaISP_AFEAdcRelatedErr_numb(58)) -> Input Conversion Subsystem/346(Inport_346)
  Harness Inputs/347(GaISP_AFEAdcRelatedErr_numb(59)) -> Input Conversion Subsystem/347(Inport_347)
  Harness Inputs/348(GaISP_AFEAdcRelatedErr_numb(60)) -> Input Conversion Subsystem/348(Inport_348)
  Harness Inputs/349(GaISP_AFEAdcRelatedErr_numb(61)) -> Input Conversion Subsystem/349(Inport_349)
  Harness Inputs/350(GaISP_AFEAdcRelatedErr_numb(62)) -> Input Conversion Subsystem/350(Inport_350)
  Harness Inputs/351(GaISP_AFEAdcRelatedErr_numb(63)) -> Input Conversion Subsystem/351(Inport_351)
  Harness Inputs/352(GaISP_AFEAdcRelatedErr_numb(64)) -> Input Conversion Subsystem/352(Inport_352)
  Harness Inputs/353(GaISP_AFEAdcRelatedErr_numb(65)) -> Input Conversion Subsystem/353(Inport_353)
  Harness Inputs/354(GaISP_AFEAdcRelatedErr_numb(66)) -> Input Conversion Subsystem/354(Inport_354)
  Harness Inputs/355(GaISP_AFEAdcRelatedErr_numb(67)) -> Input Conversion Subsystem/355(Inport_355)
  Harness Inputs/356(GaISP_AFEAdcRelatedErr_numb(68)) -> Input Conversion Subsystem/356(Inport_356)
  Harness Inputs/357(GaISP_AFEAdcRelatedErr_numb(69)) -> Input Conversion Subsystem/357(Inport_357)
  Harness Inputs/358(GaISP_AFEAdcRelatedErr_numb(70)) -> Input Conversion Subsystem/358(Inport_358)
  Harness Inputs/359(GaISP_AFEAdcRelatedErr_numb(71)) -> Input Conversion Subsystem/359(Inport_359)
  Harness Inputs/360(GaISP_AFEAdcRelatedErr_numb(72)) -> Input Conversion Subsystem/360(Inport_360)
  Harness Inputs/361(GaISP_AFEAdcRelatedErr_numb(73)) -> Input Conversion Subsystem/361(Inport_361)
  Harness Inputs/362(GaISP_AFEAdcRelatedErr_numb(74)) -> Input Conversion Subsystem/362(Inport_362)
  Harness Inputs/363(GaISP_AFEAdcRelatedErr_numb(75)) -> Input Conversion Subsystem/363(Inport_363)
  Harness Inputs/364(GaISP_AFEAdcRelatedErr_numb(76)) -> Input Conversion Subsystem/364(Inport_364)
  Harness Inputs/365(GaISP_AFEAdcRelatedErr_numb(77)) -> Input Conversion Subsystem/365(Inport_365)
  Harness Inputs/366(GaISP_AFEAdcRelatedErr_numb(78)) -> Input Conversion Subsystem/366(Inport_366)
  Harness Inputs/367(GaISP_AFEAdcRelatedErr_numb(79)) -> Input Conversion Subsystem/367(Inport_367)
  Harness Inputs/368(GaISP_AFEAdcRelatedErr_numb(80)) -> Input Conversion Subsystem/368(Inport_368)
  Harness Inputs/369(GaISP_AFEAdcRelatedErr_numb(81)) -> Input Conversion Subsystem/369(Inport_369)
  Harness Inputs/370(GaISP_AFEAdcRelatedErr_numb(82)) -> Input Conversion Subsystem/370(Inport_370)
  Harness Inputs/371(GaISP_AFEAdcRelatedErr_numb(83)) -> Input Conversion Subsystem/371(Inport_371)
  Harness Inputs/372(GaISP_AFEAdcRelatedErr_numb(84)) -> Input Conversion Subsystem/372(Inport_372)
  Harness Inputs/373(GaISP_AFEAdcRelatedErr_numb(85)) -> Input Conversion Subsystem/373(Inport_373)
  Harness Inputs/374(GaISP_AFEAdcRelatedErr_numb(86)) -> Input Conversion Subsystem/374(Inport_374)
  Harness Inputs/375(GaISP_AFEAdcRelatedErr_numb(87)) -> Input Conversion Subsystem/375(Inport_375)
  Harness Inputs/376(GaISP_AFEAdcRelatedErr_numb(88)) -> Input Conversion Subsystem/376(Inport_376)
  Harness Inputs/377(GaISP_AFEAdcRelatedErr_numb(89)) -> Input Conversion Subsystem/377(Inport_377)
  Harness Inputs/378(GaISP_AFEAdcRelatedErr_numb(90)) -> Input Conversion Subsystem/378(Inport_378)
  Harness Inputs/379(GaISP_AFEAdcRelatedErr_numb(91)) -> Input Conversion Subsystem/379(Inport_379)
  Harness Inputs/380(GaISP_AFEAdcRelatedErr_numb(92)) -> Input Conversion Subsystem/380(Inport_380)
  Harness Inputs/381(GaISP_AFEAdcRelatedErr_numb(93)) -> Input Conversion Subsystem/381(Inport_381)
  Harness Inputs/382(GaISP_AFEAdcRelatedErr_numb(94)) -> Input Conversion Subsystem/382(Inport_382)
  Harness Inputs/383(GaISP_AFEAdcRelatedErr_numb(95)) -> Input Conversion Subsystem/383(Inport_383)
  Harness Inputs/384(GaISP_AFEAdcRelatedErr_numb(96)) -> Input Conversion Subsystem/384(Inport_384)
  Harness Inputs/385(GaISP_AFEAdcRelatedErr_numb(97)) -> Input Conversion Subsystem/385(Inport_385)
  Harness Inputs/386(GaISP_AFEAdcRelatedErr_numb(98)) -> Input Conversion Subsystem/386(Inport_386)
  Harness Inputs/387(GaISP_AFEAdcRelatedErr_numb(99)) -> Input Conversion Subsystem/387(Inport_387)
  Harness Inputs/388(GaISP_AFEAdcRelatedErr_numb(100)) -> Input Conversion Subsystem/388(Inport_388)
  Harness Inputs/389(GaISP_AFEAdcRelatedErr_numb(101)) -> Input Conversion Subsystem/389(Inport_389)
  Harness Inputs/390(GaISP_AFEAdcRelatedErr_numb(102)) -> Input Conversion Subsystem/390(Inport_390)
  Harness Inputs/391(GaISP_AFEAdcRelatedErr_numb(103)) -> Input Conversion Subsystem/391(Inport_391)
  Harness Inputs/392(GaISP_AFEAdcRelatedErr_numb(104)) -> Input Conversion Subsystem/392(Inport_392)
  Harness Inputs/393(GaISP_AFEAdcRelatedErr_numb(105)) -> Input Conversion Subsystem/393(Inport_393)
  Harness Inputs/394(GaISP_AFEAdcRelatedErr_numb(106)) -> Input Conversion Subsystem/394(Inport_394)
  Harness Inputs/395(GaISP_AFEAdcRelatedErr_numb(107)) -> Input Conversion Subsystem/395(Inport_395)
  Harness Inputs/396(GaISP_AFEAdcRelatedErr_numb(108)) -> Input Conversion Subsystem/396(Inport_396)
  Harness Inputs/397(GaISP_AFEAdcRelatedErr_numb(109)) -> Input Conversion Subsystem/397(Inport_397)
  Harness Inputs/398(GaISP_AFEAdcRelatedErr_numb(110)) -> Input Conversion Subsystem/398(Inport_398)
  Harness Inputs/399(GaISP_AFEAdcRelatedErr_numb(111)) -> Input Conversion Subsystem/399(Inport_399)
  Harness Inputs/400(GaISP_AFEAdcRelatedErr_numb(112)) -> Input Conversion Subsystem/400(Inport_400)
  Harness Inputs/401(GaISP_AFEDiagModeExitErr_numb(1)) -> Input Conversion Subsystem/401(Inport_401)
  Harness Inputs/402(GaISP_AFEDiagModeExitErr_numb(2)) -> Input Conversion Subsystem/402(Inport_402)
  Harness Inputs/403(GaISP_AFEDiagModeExitErr_numb(3)) -> Input Conversion Subsystem/403(Inport_403)
  Harness Inputs/404(GaISP_AFEDiagModeExitErr_numb(4)) -> Input Conversion Subsystem/404(Inport_404)
  Harness Inputs/405(GaISP_AFEDiagModeExitErr_numb(5)) -> Input Conversion Subsystem/405(Inport_405)
  Harness Inputs/406(GaISP_AFEDiagModeExitErr_numb(6)) -> Input Conversion Subsystem/406(Inport_406)
  Harness Inputs/407(GaISP_AFEDiagModeExitErr_numb(7)) -> Input Conversion Subsystem/407(Inport_407)
  Harness Inputs/408(GaISP_AFEDiagModeExitErr_numb(8)) -> Input Conversion Subsystem/408(Inport_408)
  Harness Inputs/409(GaISP_AFEOtherErr_numb(1)) -> Input Conversion Subsystem/409(Inport_409)
  Harness Inputs/410(GaISP_AFEOtherErr_numb(2)) -> Input Conversion Subsystem/410(Inport_410)
  Harness Inputs/411(GaISP_AFEOtherErr_numb(3)) -> Input Conversion Subsystem/411(Inport_411)
  Harness Inputs/412(GaISP_AFEOtherErr_numb(4)) -> Input Conversion Subsystem/412(Inport_412)
  Harness Inputs/413(GaISP_AFEOtherErr_numb(5)) -> Input Conversion Subsystem/413(Inport_413)
  Harness Inputs/414(GaISP_AFEOtherErr_numb(6)) -> Input Conversion Subsystem/414(Inport_414)
  Harness Inputs/415(GaISP_AFEOtherErr_numb(7)) -> Input Conversion Subsystem/415(Inport_415)
  Harness Inputs/416(GaISP_AFEOtherErr_numb(8)) -> Input Conversion Subsystem/416(Inport_416)
  Harness Inputs/417(GaISP_AFESampleErr_numb(1)) -> Input Conversion Subsystem/417(Inport_417)
  Harness Inputs/418(GaISP_AFESampleErr_numb(2)) -> Input Conversion Subsystem/418(Inport_418)
  Harness Inputs/419(GaISP_AFESampleErr_numb(3)) -> Input Conversion Subsystem/419(Inport_419)
  Harness Inputs/420(GaISP_AFESampleErr_numb(4)) -> Input Conversion Subsystem/420(Inport_420)
  Harness Inputs/421(GaISP_AFESampleErr_numb(5)) -> Input Conversion Subsystem/421(Inport_421)
  Harness Inputs/422(GaISP_AFESampleErr_numb(6)) -> Input Conversion Subsystem/422(Inport_422)
  Harness Inputs/423(GaISP_AFESampleErr_numb(7)) -> Input Conversion Subsystem/423(Inport_423)
  Harness Inputs/424(GaISP_AFESampleErr_numb(8)) -> Input Conversion Subsystem/424(Inport_424)
  Harness Inputs/425(GeUDS_CapSel_enum) -> Input Conversion Subsystem/425(Inport_425)
  Output Conversion Subsystem/1(Outport_1) -> GaCFM_AFEComLost_flg/1
  Output Conversion Subsystem/2(Outport_2) -> GaCFM_AFECellVoltUpdErr_flg/1
  Output Conversion Subsystem/3(Outport_3) -> GaCFM_AFECellTempUpdErr_flg/1
  Output Conversion Subsystem/4(Outport_4) -> GaCFM_AFECellVoltLineOpen_flg/1
  Output Conversion Subsystem/5(Outport_5) -> GaCFM_AFEGpioLineOpen_flg/1
  Output Conversion Subsystem/6(Outport_6) -> GaCFM_AFEAdcRelatedErr_flg/1
  Output Conversion Subsystem/7(Outport_7) -> GaCFM_AFEDiagModeExitErr_flg/1
  Output Conversion Subsystem/8(Outport_8) -> GaCFM_AFEOtherErr_flg/1
  Output Conversion Subsystem/9(Outport_9) -> GaCFM_AFESampleErr_flg/1
  Input Conversion Subsystem/1(Outport_1) -> CFM_MIL/1
  Input Conversion Subsystem/2(Outport_2) -> CFM_MIL/2
  Input Conversion Subsystem/3(Outport_3) -> CFM_MIL/3
  Input Conversion Subsystem/4(Outport_4) -> CFM_MIL/4
  Input Conversion Subsystem/5(Outport_5) -> CFM_MIL/5
  Input Conversion Subsystem/6(Outport_6) -> CFM_MIL/6
  Input Conversion Subsystem/7(Outport_7) -> CFM_MIL/7
  Input Conversion Subsystem/8(Outport_8) -> CFM_MIL/8
  Input Conversion Subsystem/9(Outport_9) -> CFM_MIL/9
  Input Conversion Subsystem/10(Outport_10) -> CFM_MIL/10
  CFM_MIL/1 -> Output Conversion Subsystem/1(Inport_1)
  CFM_MIL/2 -> Output Conversion Subsystem/2(Inport_2)
  CFM_MIL/3 -> Output Conversion Subsystem/3(Inport_3)
  CFM_MIL/4 -> Output Conversion Subsystem/4(Inport_4)
  CFM_MIL/5 -> Output Conversion Subsystem/5(Inport_5)
  CFM_MIL/6 -> Output Conversion Subsystem/6(Inport_6)
  CFM_MIL/7 -> Output Conversion Subsystem/7(Inport_7)
  CFM_MIL/8 -> Output Conversion Subsystem/8(Inport_8)
  CFM_MIL/9 -> Output Conversion Subsystem/9(Inport_9)
